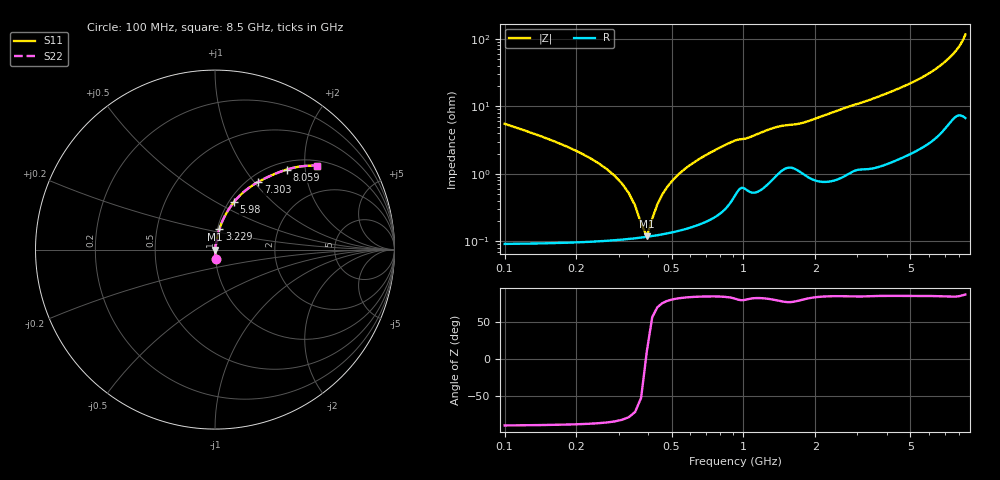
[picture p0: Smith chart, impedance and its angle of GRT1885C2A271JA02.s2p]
!Murata Part Number: GRT1885C2A271JA02
!These Parameters are Measured in Series Mode Connection
!Data Generated on Jun 19, 2026
!  o--ll--o
!Port1  Port2
!  o------o
!Operation Temp=25[degC], DC Bias Voltage=0[V]
!Freq. Start=100[MHz] Stop=9[GHz] 401[Steps]
# Hz S RI R 50
!Freq.(Hz) S11(Real) S11(Imag) S21(Real) S21(Imag) S12(Real) S12(Imag) S22(Real) S22(Imag)
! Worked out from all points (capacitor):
!   401 points, 100 MHz to 8.5 GHz, reference 50 ohm
!   read as one part in series: C = 270 pF near 142 MHz
!   lowest |Z| = 119 mohm at 394 MHz (marker M1)
!   series resonance near 391.3 MHz, so ESL is about 610 pH
!   S11 on the Smith chart (normalised r, x): 100 MHz: 1.00, -0.11; 3.229 GHz: 1.02, +0.24; 5.98 GHz: 1.06, +0.61; 7.303 GHz: 1.11, +1.05; 8.059 GHz: 1.15, +1.60; 8.5 GHz: 1.13, +2.32
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1e8  0.00394 -0.0549  0.9961 0.0549  0.9961 0.0549  0.00394 -0.0549
2.68e8  0.00115 -0.0117  0.9988 0.0117  0.9988 0.0117  0.00115 -0.0117
3.1e8  0.00111 -0.00709  0.9989 0.00709  0.9989 0.00709  0.00111 -0.00709
3.52e8  0.00112 -0.0032  0.9989 0.0032  0.9989 0.0032  0.00112 -0.0032
3.73e8  0.00114 -0.00144  0.9989 0.00144  0.9989 0.00144  0.00114 -0.00144
3.94e8  0.00117 0.000216  0.9988 -0.000216  0.9988 -0.000216  0.00117 0.000216
4.15e8  0.0012 0.00179  0.9988 -0.00179  0.9988 -0.00179  0.0012 0.00179
4.78e8  0.00134 0.00613  0.9987 -0.00613  0.9987 -0.00613  0.00134 0.00613
5.2e8  0.00147 0.00879  0.9985 -0.00879  0.9985 -0.00879  0.00147 0.00879
6.04e8  0.0018 0.0137  0.9982 -0.0137  0.9982 -0.0137  0.0018 0.0137
7.09e8  0.00238 0.0195  0.9976 -0.0195  0.9976 -0.0195  0.00238 0.0195
9.19e8  0.00559 0.0304  0.9944 -0.0304  0.9944 -0.0304  0.00559 0.0304
1.507e9  0.0144 0.0497  0.9856 -0.0497  0.9856 -0.0497  0.0144 0.0497
2.914e9  0.0214 0.1013  0.9786 -0.1013  0.9786 -0.1013  0.0214 0.1013
3.229e9  0.0247 0.1133  0.9753 -0.1133  0.9753 -0.1133  0.0247 0.1133
4.3e9  0.043 0.163  0.957 -0.163  0.957 -0.163  0.043 0.163
5.707e9  0.0917 0.2466  0.9083 -0.2466  0.9083 -0.2466  0.0917 0.2466
5.98e9  0.107 0.2666  0.893 -0.2666  0.893 -0.2666  0.107 0.2666
7.114e9  0.2146 0.3616  0.7854 -0.3616  0.7854 -0.3616  0.2146 0.3616
7.303e9  0.2422 0.3781  0.7578 -0.3781  0.7578 -0.3781  0.2422 0.3781
8.059e9  0.4003 0.4461  0.5997 -0.4461  0.5997 -0.4461  0.4003 0.4461
8.5e9  0.5707 0.4669  0.4293 -0.4669  0.4293 -0.4669  0.5707 0.4669
